(* Logix 5000 Rung export; software revision 24.00 *)

TYPE SNAPP_CONTROL_22 :
STRUCT
   Reserved_0_0 : BOOL;
   Trigger : BOOL;
   Reserved_0_2 : BOOL;
   InspectionResultsAck : BOOL;
   ExecuteCommand : BOOL;
   Reserved_0_5 : BOOL;
   Reserved_0_6 : BOOL;
   Reserved_0_7 : BOOL;
   Reserved_Byte1 : SINT;
   Reserved_2_0 : BOOL;
   Reserved_2_1 : BOOL;
   ClearError : BOOL;
   Reserved_2_3 : BOOL;
   Reserved_2_4 : BOOL;
   Reserved_2_5 : BOOL;
   Reserved_2_6 : BOOL;
   Reserved_2_7 : BOOL;
   Reserved_3_0 : BOOL;
   Reserved_3_1 : BOOL;
   Reserved_3_2 : BOOL;
   Reserved_3_3 : BOOL;
   Reserved_3_4 : BOOL;
   Reserved_3_5 : BOOL;
   Reserved_3_6 : BOOL;
   Reserved_3_7 : BOOL;
   CommandID : INT;
   Reserved_Bytes6and7 : INT;
END_STRUCT
END_TYPE

TYPE SNAPP_IN_13 :
STRUCT
   Status : SNAPP_STAT_IN_13;
   InspectionResults : SNAPP_RESULTS_13;
END_STRUCT
END_TYPE

TYPE SNAPP_STAT_IN_13 :
STRUCT
   TriggerReady : BOOL;
   TriggerAck : BOOL;
   Reserved_0_2 : BOOL;
   AcqError : BOOL;
   Reserved_0_4 : BOOL;
   Reserved_0_5 : BOOL;
   Reserved_0_6 : BOOL;
   Online : BOOL;
   Reserved_1_0 : BOOL;
   InspectionCompleted : BOOL;
   Reserved_1_2 : BOOL;
   ResultsValid : BOOL;
   CommandExecuting : BOOL;
   CommandCompleted : BOOL;
   CommandFailed : BOOL;
   Error : BOOL;
   Reserved_2_0 : BOOL;
   Reserved_2_1 : BOOL;
   Reserved_2_2 : BOOL;
   Reserved_2_3 : BOOL;
   InspectionPass : BOOL;
   Reserved_2_5 : BOOL;
   Reserved_2_6 : BOOL;
   Reserved_2_7 : BOOL;
   Reserved_3_0 : BOOL;
   Reserved_3_1 : BOOL;
   Reserved_3_2 : BOOL;
   Reserved_3_3 : BOOL;
   Reserved_3_4 : BOOL;
   Reserved_3_5 : BOOL;
   Reserved_3_6 : BOOL;
   Reserved_3_7 : BOOL;
   ErrorID : INT;
   Reserved_Bytes_6_7 : INT;
   CurrentProgramID : INT;
   AcquisitionID : INT;
   InspectionID : INT;
   Reserved_Bytes_14_15 : INT;
END_STRUCT
END_TYPE

TYPE SNAPP_RESULTS_13 :   // Inspection Results from Sensor
STRUCT
   PayloadVersion : SINT;
   ApplicationType : SINT;   // 0=Error, 1=Anomaly Detection, 2=Binary Classifier, 3=4-Class Binary Classifier, 4...255=Reserved
   Program : SINT;
   InspectionStatusCode : SINT;   // 0=Inspection Valid, 1=Sensor Untrained, 2=Fixture Not Found, 3=ROI Outside Image, 4...255=Reserved
   IdentifiedClassEnum : SINT;   // Anomaly: 0=Reserved, 1=OK, 2=NG, 3-254=Reserved, 255=Error
   IdentifiedClassConfidence : SINT;
   ClassName : SINT[474];
END_STRUCT
END_TYPE

TYPE SNAPP_OUT_22 :
STRUCT
   Control : SNAPP_CONTROL_22;
END_STRUCT
END_TYPE

VAR_GLOBAL   (* controller tags *)
   SNAPP:I1 : _02A6:IS28XX_XX_F1075143:I:0;
   SNAPPManualTrigger : BOOL;
   SNAPP2800_Out : SNAPP_OUT_22 := (Control.CommandID := 1);
   SNAPP:O1 : _02A6:IS28XX_XX_DD7B81FB:O:0 := (Data[0] := 8, Data[4] := 21);
   TimerTriggerSNAPP : TIMER := (PRE := 500);
   SNAPP2800_In : SNAPP_IN_13;
   SNAPPAutoTrigger : BOOL;
END_VAR

PROGRAM MainProgram

ROUTINE SNAPPky   (* ladder *)
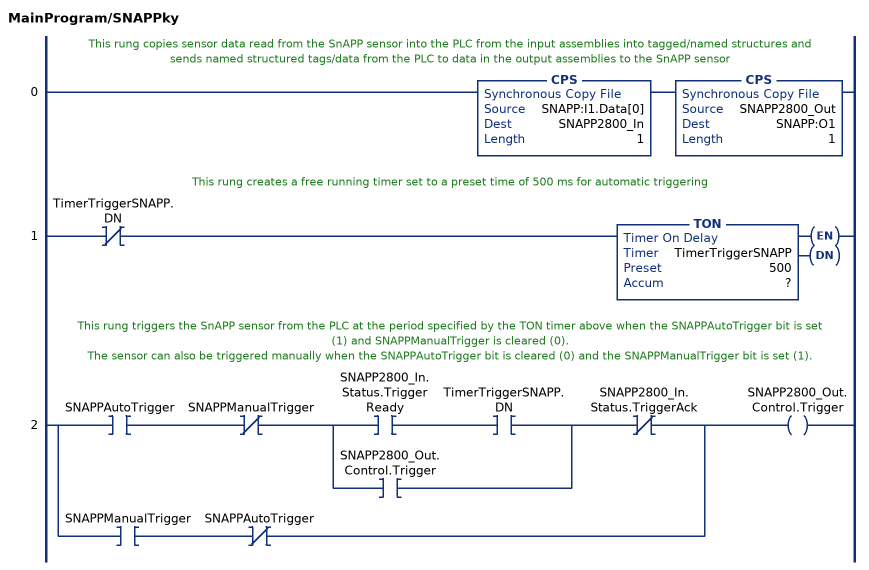
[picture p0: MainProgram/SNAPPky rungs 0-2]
   // This rung copies sensor data read from the SnAPP sensor into the PLC from the input assemblies into tagged/named structures and sends named structured tags/data from the PLC to data in the output assemblies to the SnAPP sensor
   0: CPS(SNAPP:I1.Data[0],SNAPP2800_In,1)CPS(SNAPP2800_Out,SNAPP:O1,1);
   // This rung creates a free running timer set to a preset time of 500 ms for automatic triggering
   1: XIO(TimerTriggerSNAPP.DN)TON(TimerTriggerSNAPP,?,?);
   // This rung triggers the SnAPP sensor from the PLC at the period specified by the TON timer above when the SNAPPAutoTrigger bit is set (1) and SNAPPManualTrigger is cleared (0).
   // The sensor can also be triggered manually when the SNAPPAutoTrigger bit is cleared (0) and the SNAPPManualTrigger bit is set (1).
   2: [XIC(SNAPPAutoTrigger) XIO(SNAPPManualTrigger) [XIC(SNAPP2800_In.Status.TriggerReady) XIC(TimerTriggerSNAPP.DN) ,XIC(SNAPP2800_Out.Control.Trigger) ] XIO(SNAPP2800_In.Status.TriggerAck) ,XIC(SNAPPManualTrigger) XIO(SNAPPAutoTrigger) ]OTE(SNAPP2800_Out.Control.Trigger);
END_ROUTINE
END_PROGRAM
